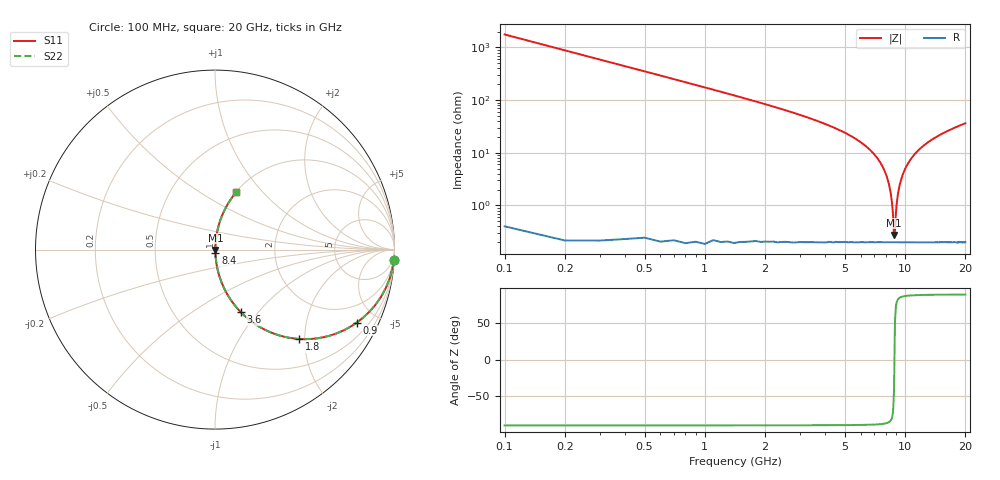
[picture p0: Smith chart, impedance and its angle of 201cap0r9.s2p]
! AVX Thin Film Operation		Date: May 2007
! Description: Accu-P® Series, Thin Film, SMD, RF Capacitor
! Part Number: 02013J0R9ABS
! 50 MHz  -  20.05 GHz
! Serial Measurements
# hz S db R 50
!	S11		S21		S12		S22
!	dB	Phase	dB	Phase	dB	Phase	dB	Phase
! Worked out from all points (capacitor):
!   200 points, 100 MHz to 20 GHz, reference 50 ohm
!   read as one part in series: C = 900 fF near 200 MHz
!   lowest |Z| = 276 mohm at 8.8 GHz (marker M1)
!   series resonance near 8.842 GHz, so ESL is about 360 pH
!   S11 on the Smith chart (normalised r, x): 100 MHz: 1, -35; 900 MHz: 1.00, -3.89; 1.8 GHz: 1.00, -1.88; 3.6 GHz: 1.00, -0.82; 8.4 GHz: 1.00, -0.04; 20 GHz: 1.00, +0.73
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1e8  -0.01 -3.2  -24.96 86.8  -24.96 86.8  -0.01 -3.2
2e8  -0.06 -6.5  -18.98 83.5  -18.98 83.5  -0.06 -6.5
4e8  -0.22 -12.8  -13.11 77.2  -13.11 77.2  -0.22 -12.8
9e8  -1.02 -27.2  -6.80 62.7  -6.80 62.7  -1.02 -27.2
1.8e9  -3.29 -46.6  -2.77 43.2  -2.77 43.2  -3.29 -46.6
3.5e9  -8.15 -66.7  -0.74 23.0  -0.74 23.0  -8.15 -66.7
3.6e9  -8.44 -67.5  -0.69 22.2  -0.69 22.2  -8.44 -67.5
6.8e9  -19.54 -82.9  -0.07 6.1  -0.07 6.1  -19.54 -82.9
7.8e9  -25.99 -84.8  -0.03 2.9  -0.03 2.9  -25.99 -84.8
8.4e9  -33.74 -83.3  -0.02 1.2  -0.02 1.2  -33.74 -83.3
8.6e9  -38.97 -79.2  -0.02 0.6  -0.02 0.6  -38.97 -79.2
8.7e9  -43.40 -72.5  -0.02 0.4  -0.02 0.4  -43.40 -72.5
8.8e9  -51.20 -43.4  -0.02 0.1  -0.02 0.1  -51.20 -43.4
8.9e9  -49.66 52.5  -0.02 -0.1  -0.02 -0.1  -49.66 52.5
9e9  -42.67 73.8  -0.02 -0.4  -0.02 -0.4  -42.67 73.8
9.1e9  -38.67 79.5  -0.02 -0.7  -0.02 -0.7  -38.67 79.5
9.3e9  -33.86 83.2  -0.02 -1.2  -0.02 -1.2  -33.86 83.2
1.01e10  -25.48 84.8  -0.03 -3.0  -0.03 -3.0  -25.48 84.8
1.14e10  -19.83 83.0  -0.06 -5.9  -0.06 -5.9  -19.83 83.0
1.34e10  -15.48 79.6  -0.14 -9.7  -0.14 -9.7  -15.48 79.6
1.67e10  -11.64 74.4  -0.33 -15.2  -0.33 -15.2  -11.64 74.4
2e10  -9.33 69.7  -0.56 -20.0  -0.56 -20.0  -9.33 69.7
